INTERFACE I_Device

PROPERTY DeviceId : UDINT
END_PROPERTY

PROPERTY IsOnline : BOOL
END_PROPERTY

METHOD Initialize : BOOL
VAR_INPUT
    nId : UDINT;
END_VAR
END_METHOD

METHOD Execute : BOOL
END_METHOD

METHOD GetStatus : INT
END_METHOD

END_INTERFACE
